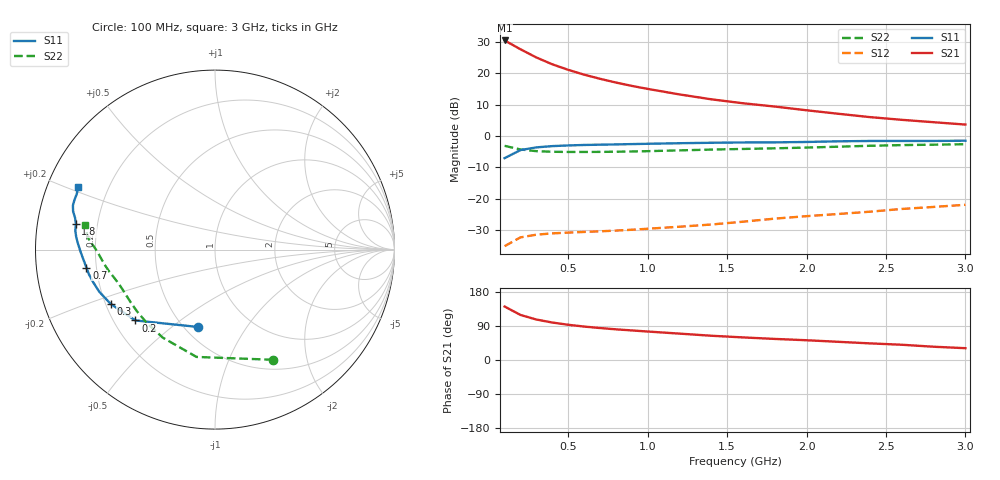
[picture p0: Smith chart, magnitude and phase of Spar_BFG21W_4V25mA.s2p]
! Filename: 425bfg21.001
! Title: BFG21W
! Bias: Vce=4V; Ic=25mA
! Company: NXP Semiconductors NL
! User: Quality&Reliability T&D
! Measure time: 10 Nov 1999 / 11:45:05
#  MHz  S  MA  R 50
! Freq  S11  S21  S12  S22  :
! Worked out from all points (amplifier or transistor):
!   20 points, 100 MHz to 3 GHz, reference 50 ohm
!   highest |S21| = 30.4 dB at 100 MHz (marker M1)
!   |S21| within 3 dB of that: start of sweep to 207.1 MHz
!   unconditionally stable (mu >= 1): 1.119 GHz to end of sweep
!   at 400 MHz: K = 0.49, MSG = 27.0 dB, |S12| = -31.1 dB
!   at 1.2 GHz: K = 1.04, MAG = 20.0 dB, |S12| = -29.0 dB
!   at 3 GHz: K = 1.05, MAG = 11.4 dB, |S12| = -22.0 dB
!   S11 on the Smith chart (normalised r, x): 100 MHz: 0.58, -0.62; 200 MHz: 0.29, -0.35; 300 MHz: 0.22, -0.23; 700 MHz: 0.16, -0.07; 1.8 GHz: 0.12, +0.09; 3 GHz: 0.09, +0.22
100  0.4414 -102.5  33.28 141.1  0.0174 46.6  0.6936 -62.2
200  0.5935 -138.3  24.07 118.9  0.02405 35.9  0.6068 -99.8
300  0.6554 -152.5  17.8 106.8  0.02655 31.3  0.5703 -120.7
400  0.6864 -160.0  13.87 98.9  0.02784 30.2  0.5578 -133.3
500  0.7037 -165.3  11.32 93.0  0.02864 30.6  0.5541 -141.6
600  0.716 -169.0  9.482 88.3  0.02935 32.1  0.5539 -147.3
700  0.7235 -172.0  8.143 84.4  0.03002 34.3  0.5554 -151.7
800  0.7309 -174.5  7.099 80.9  0.03084 36.9  0.5586 -155.2
900  0.7396 -176.8  6.273 78.0  0.0318 39.9  0.5638 -158.2
1000  0.7479 -178.8  5.618 75.1  0.03299 42.5  0.5703 -160.9
1200  0.7636 177.7  4.587 69.6  0.03554 47.7  0.5871 -165.3
1400  0.7763 174.9  3.834 64.0  0.03855 52.3  0.6043 -168.8
1600  0.7853 172.3  3.315 59.6  0.04275 56.6  0.6186 -171.8
1800  0.7882 169.5  2.936 55.6  0.04786 60.1  0.6333 -174.9
2000  0.7994 167.2  2.56 52.1  0.05237 63.2  0.6507 -178.2
2200  0.819 164.9  2.252 48.0  0.05674 65.3  0.6721 178.8
2400  0.8291 162.7  1.991 43.8  0.06177 66.4  0.6951 176.5
2600  0.8305 160.6  1.803 40.2  0.06828 66.8  0.7127 174.4
2800  0.8303 158.1  1.652 35.0  0.07352 66.2  0.7238 172.0
3000  0.8373 155.4  1.515 31.2  0.07958 66.2  0.7355 169.1
